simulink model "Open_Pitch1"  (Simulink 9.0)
settings: Solver=ode45  StartTime=0.0  StopTime=150  RelTol=1e-3  EnableMultiTasking=on
InitFcn:
  | r2d= 180/pi; d2r=pi/180;
  | [Ap,Bp,Cp,Dp]= vehi_pitch;                    % Load the Pitch Analysis Model
  | load Kc.mat -ascii
undefined symbols (not defined in the file or in its folder): Ap, Bp, Cp, Dp, Kc

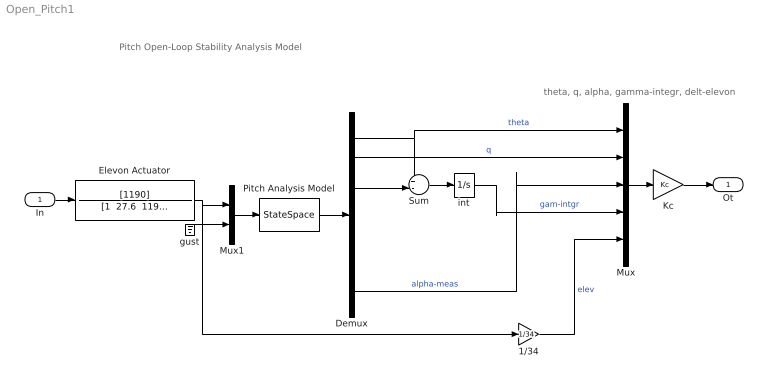
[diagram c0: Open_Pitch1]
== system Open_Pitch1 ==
  note: Pitch Open-Loop Stability Analysis Model
  note: theta, q, alpha, gamma-integr, delt-elevon
  In : Inport
  1/34 : Gain  Gain=1/34
  Demux : Demux  Outputs=7
  Elevon Actuator : TransferFcn  Numerator=[1190]  Denominator="[1  27.6  1190]"
  Kc : Gain  Gain=Kc  Multiplication=Matrix(K*u)
  Mux : Mux  Inputs=5
  Mux1 : Mux  Inputs=2
  Pitch Analysis Model : StateSpace  A=Ap  B=Bp  C=Cp  D=Dp  InitialCondition=0
  Sum : Sum  Inputs=+-|
  gust : Ground
  int : Integrator
  Ot : Outport
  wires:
  Demux/1 -> Mux/1, Sum/1  "theta"
  Mux/1 -> Kc/1
  1/34/1 -> Mux/5  "elev"
  int/1 -> Mux/4  "gam-intgr"
  Sum/1 -> int/1
  Kc/1 -> Ot/1
  Mux1/1 -> Pitch Analysis Model/1
  In/1 -> Elevon Actuator/1
  gust/1 -> Mux1/2
  Elevon Actuator/1 -> 1/34/1, Mux1/1
  Pitch Analysis Model/1 -> Demux/1
  Demux/2 -> Mux/2  "q"
  Demux/3 -> Sum/2
  Demux/7 -> Mux/3  "alpha-meas"
